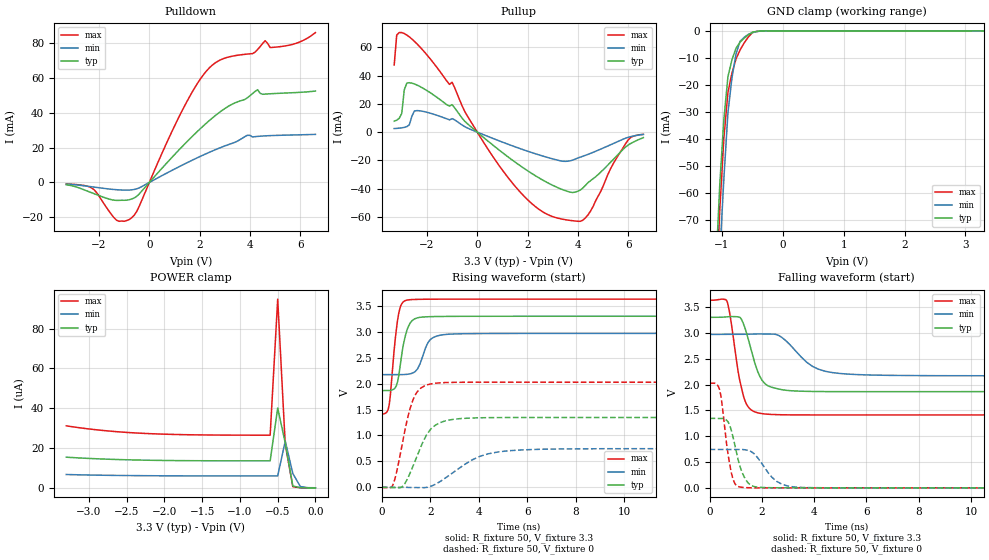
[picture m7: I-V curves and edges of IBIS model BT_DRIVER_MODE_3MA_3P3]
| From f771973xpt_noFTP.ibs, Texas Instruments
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|   Model Cell BT_DRIVER_MODE_3MA_3P3
|BT_DRIVER_MODE_3MA_3P3
[Model]   BT_DRIVER_MODE_3MA_3P3
Model_type   I/O
Polarity   Non-Inverting
Enable   Active-Low
Vinl =  0.8
Vinh =  2
Cref =  15.0000pF
Rref =  100.0000M
Vref =  0V
Vmeas =  1.65
C_comp   3.98845p   2.03906p   4.55356p
[Model Spec]
Vinl   0.8   0.8   0.8
Vinh   2   2   2
[Temperature Range]   25   155   -40
[Voltage Range]   3.3   2.97   3.63
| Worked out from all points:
|   slope of the pulldown table from 0 to 0.495 V, typ, clamps not added: 61.7 ohm
|   slope of the pullup table from 0 to 0.495 V, typ, clamps not added: 67.2 ohm
|   GND clamp passes 1 mA (typ) near -0.53 V on its own axis
|   rising waveform, R_fixture 50, V_fixture 3.3: 20-80 % time 326ps typ, 410ps min, 271ps max; typ from 1.87 V to 3.3 V
|   rising waveform, R_fixture 50, V_fixture 0: 20-80 % time 783ps typ, 1.51ns min, 573ps max; typ from 0 V to 1.34 V
|   falling waveform, R_fixture 50, V_fixture 3.3: 20-80 % time 525ps typ, 1.02ns min, 426ps max; typ from 3.3 V to 1.86 V
|   falling waveform, R_fixture 50, V_fixture 0: 20-80 % time 420ps typ, 693ps min, 312ps max; typ from 1.34 V to 0 V
| Nom Voltages:
|   BIASFET=3.3, VDD=1.2, VDDS=3.3, VSS=0
| Min Voltages:
|   BIASFET=2.97, VDD=1.08, VDDS=2.97, VSS=0
| Max Voltages:
|   BIASFET=3.63, VDD=1.32, VDDS=3.63, VSS=0
[POWER_clamp]
|   voltage   I(typ)   I(min)   I(max)
-3.3V     15.41uA    6.707uA    31.17uA
-2.8V     14.47uA    6.332uA    28.78uA
-2.2V     13.87uA    6.102uA    27.25uA
-1.6V     13.64uA    6.016uA    26.64uA
-600mV    13.58uA    5.99uA     26.46uA
-500mV    40.13uA    5.991uA    94.83uA
-400mV    22.54uA    23.52uA    21.76uA
-300mV    969.1nA    7.216uA    616.4nA
-200mV    29.93nA    661.1nA    11.88nA
0V        1.388nA    48.32nA    1.243nA
[Pulldown]
|   voltage   I(typ)   I(min)   I(max)
-3.3V     -1.368mA   -936.2uA   -859.1uA
-2.3V     -5.876mA   -2.477mA   -3.094mA
-1.3V     -10.31mA   -4.18mA    -21.72mA
-800mV    -9.945mA   -4.384mA   -21.31mA
-500mV    -7.961mA   -3.661mA   -16.65mA
1.4V      21.97mA    10.6mA     43.88mA
2.4V      35.71mA    17.39mA    65.97mA
4.3V      53.2mA     26.41mA    76.22mA
4.6V      50.69mA    26.72mA    81.32mA
4.8V      50.87mA    26.86mA    77.39mA
5.4V      51.3mA     27.13mA    78.32mA
6.6V      52.45mA    27.57mA    85.99mA
[Pullup]
|   voltage   I(typ)   I(min)   I(max)
-3.3V     7.739mA    2.523mA    47.63mA
-3.2V     8.473mA    2.639mA    68.85mA
-3V       13.28mA    3.02mA     70.54mA
-2.9V     29.97mA    3.344mA    69.86mA
-2.8V     34.69mA    3.876mA    68.8mA
-2.5V     34.14mA    14.95mA    64.38mA
-1V       19.46mA    9.547mA    35.34mA
1.3V      -18.59mA   -9.091mA   -33.95mA
3.1V      -38.57mA   -19.45mA   -60.48mA
4.3V      -37.72mA   -16.43mA   -60.74mA
6V        -9.124mA   -3.659mA   -5.434mA
6.6V      -3.896mA   -1.629mA   -1.546mA
[GND_clamp]
|   voltage   I(typ)   I(min)   I(max)
-3.3V     -1.746A    -1.481A    -2.454A
-1.1V     -88.72mA   -114.8mA   -101.4mA
-1.033V   -56.66mA   -82.94mA   -65.99mA
-966.7mV  -32.75mA   -54.79mA   -39.79mA
-900mV    -16.98mA   -30.37mA   -22.81mA
-833.3mV  -10.67mA   -17.32mA   -15.58mA
-766.7mV  -6.402mA   -8.477mA   -10.34mA
-700mV    -4.171mA   -3.846mA   -7.085mA
-566.7mV  -1.511mA   -1.331mA   -2.329mA
-500mV    -537.7uA   -639.3uA   -683uA
-300mV    -1.439uA   -12.56uA   -707.1nA
3.3V      1.388nA    14.18uA    1.029nA
[Ramp]
| variable   typ   min   max
dV/dt_f 0.87243134/0.53137713n 0.48603643/1.0377786n   1.344851/0.42962575n
dV/dt_r 0.81373668/0.78906954n 0.45222846/1.5290324n  1.2226949/0.57631885n
R_load = 50
[Rising Waveform]
R_fixture = 50
V_fixture = 3.3
V_fixture_min = 2.97
V_fixture_max = 3.63
|   time   V(typ)   V(min)   V(max)
0s        1.866V     2.173V     1.413V
210.5ps   1.866V     2.173V     1.452V
308.7ps   1.868V     2.173V     1.593V
599.8ps   1.954V     2.173V     3.032V
785.8ps   2.43V      2.173V     3.504V
1.038ns   3.027V     2.179V     3.611V
1.48ns    3.27V      2.287V     3.626V
1.977ns   3.291V     2.834V     3.629V
2.72ns    3.297V     2.952V     3.63V
20.03ns   3.3V       2.97V      3.63V
[Rising Waveform]
R_fixture = 50
V_fixture = 0
V_fixture_min = 0
V_fixture_max = 0
|   time   V(typ)   V(min)   V(max)
0s        0V         0V         0V
462.7ps   -4.838mV   0V         46.66mV
875.1ps   24.7mV     0V         904.1mV
1.165ns   267.9mV    -3.134mV   1.51V
1.385ns   519.6mV    -5.293mV   1.783V
2.018ns   1.12V      19.39mV    1.994V
2.732ns   1.294V     214.4mV    2.022V
4.056ns   1.341V     598.4mV    2.027V
5.234ns   1.346V     705.2mV    2.027V
20.01ns   1.345V     744.3mV    2.026V
[Falling Waveform]
R_fixture = 50
V_fixture = 3.3
V_fixture_min = 2.97
V_fixture_max = 3.63
|   time   V(typ)   V(min)   V(max)
0s        3.3V       2.97V      3.63V
667.3ps   3.31V      2.97V      3.606V
1.125ns   3.308V     2.97V      2.146V
1.312ns   3.151V     2.972V     1.745V
1.507ns   2.821V     2.975V     1.546V
1.894ns   2.187V     2.979V     1.446V
2.726ns   1.903V     2.923V     1.415V
3.935ns   1.866V     2.351V     1.411V
4.973ns   1.862V     2.214V     1.411V
20.03ns   1.865V     2.171V     1.413V
[Falling Waveform]
R_fixture = 50
V_fixture = 0
V_fixture_min = 0
V_fixture_max = 0
|   time   V(typ)   V(min)   V(max)
0s        1.344V     743.3mV    2.026V
374ps     1.345V     743.3mV    1.909V
468ps     1.344V     743.3mV    1.647V
646.2ps   1.31V      743.3mV    856.9mV
833.1ps   1.103V     743.4mV    286.3mV
1.145ns   440.3mV    743.8mV    17.02mV
1.667ns   30.42mV    674.8mV    0V
2.554ns   0V         128.8mV    0V
3.208ns   0V         18.32mV    0V
20.01ns   0V         0V         0V
